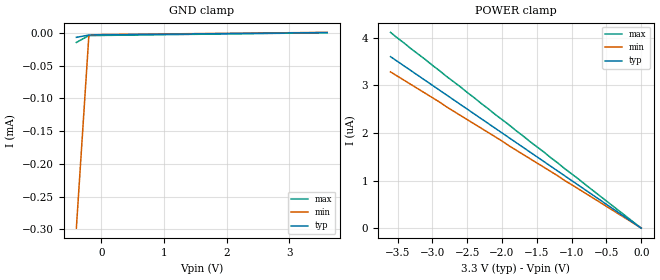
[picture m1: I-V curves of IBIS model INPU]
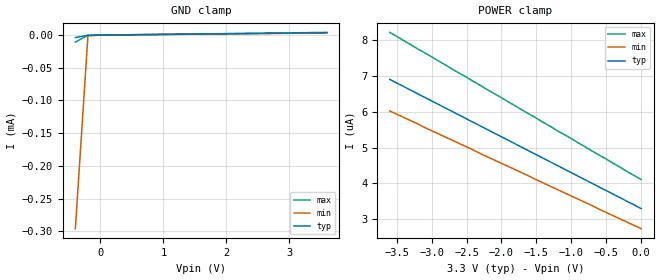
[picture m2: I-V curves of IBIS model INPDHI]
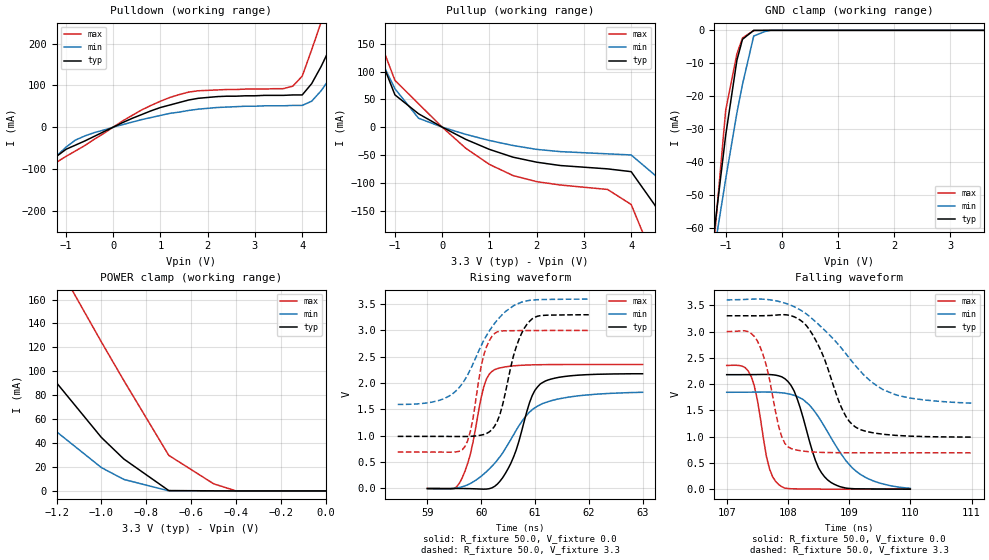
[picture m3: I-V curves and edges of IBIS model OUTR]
|   Texas Instruments Incorporated
|   Data Transmissions Products
|   IBIS Model for ISO723x4x
|   16DW SOIC Package
[IBIS Ver]   3.2
[Comment char]   |_char
[File name]   iso35.ibs
[File Rev]   1.0
[Date]   08July08
[Source]   File originated at Texas Instruments Incorporated.
   Data Transmission Products Group.
[Notes]
[Disclaimer]
(C) Copyright Texas Instruments Incorporated 2002
   All rights reserved
  Texas Instruments Incorporated hereby grants the user of this IBIS
model a non-exclusive, nontransferable license to use this IBIS model
under the following terms.  Before using this IBIS model, the user
should read this license.  If the user does not accept these terms,
the IBIS model should be returned to Texas Instruments within 30 days.
  The user is granted this license only to use the IBIS model and
is not granted rights to sell, load, rent, lease or license the IBIS
model in whole or in part, or in modified form to anyone other than
user.  User may modify the IBIS model to suit its specific applications
but rights to derivative works and such modifications shall belong to
Texas Instruments.
  This IBIS model is provided on an "AS IS" basis and Texas Instruments
makes absolutely no warranty with respect to the information contained
herein.  TEXAS INSTRUMENTS DISCLAIMS AND CUSTOMER WAIVES ALL WARRANTIES,
EXPRESS OR IMPLIED, INCLUDING WARRANTIES OF MERCHANTABILITY OR FITNESS
FOR A PARTICULAR PURPOSE. The entire risk as to quality and performance
is with the Customer. ACCORDINGLY, IN NO EVENT SHALL THE COMPANY BE LIABLE
FOR ANY DAMAGES, WHETHER IN CONTRACT OR TORT,INCLUDING ANY LOST PROFITS
OR OTHER INCIDENTAL, CONSEQUENTIAL, EXEMPLARY, OR PUNITIVE DAMAGES ARISING
OUT OF THE USE OR APPLICATION OF THE IBIS model provided in this package.
Further, Texas Instruments reserves the right to discontinue or make changes
without notice to any product herein to improve reliability, function, or
design. Texas Instruments does not convey any license under patent rights
or any other intellectual property rights, including those of third parties.
Contact Texas Instruments at ATTN:DATA TRANSMISSIONS
[Copyright]   Copyright 2002, Texas Instruments, All Rights Reserved
[Component]   ISO35DW
[Manufacturer]  Texas Instruments Incorporated
[Package]
|   typ   min   max
R_pkg   0.04817   0.03432   0.09530
L_pkg   2.4595nH   1.6904nH   4.7034nH
C_pkg   0.847pF   0.428pF   1.397pF
[Pin]   signal_name   model_name   R_pin   L_pin   C_pin
1   VCC1   POWER   0.03455  3.39778n  0.89677p
2   GND1   GND   0.03432  3.12613n  0.84706p
3   R   OUTR   0.04265  1.85523n  0.57831p
4   REB   INPU   0.03948  1.69049n  0.59300p
5   DE   INPDHI   0.03943  1.70546n  0.55709p
6   D   INPU   0.04257  1.86953n  0.56379p
7   GND1   GND   0.04783  1.99000n  0.60148p
8   GND1   GND   0.03740  4.70338n  1.39696p
9   GND2   GND   0.03763  4.61305n  1.39587p
10   GND2   GND   0.04703  2.01514n  0.58483p
11   Y   DRVR   0.07132  2.45946n  0.43321p
12   Z   DRVR   0.06147  2.13194n  0.42769p
13   B   REC   0.07288  2.39260n  0.48001p
14   A   REC   0.09530  3.03704n  0.47622p
15   GND2   GND   0.04817  4.23145n  0.93567p
16   VCC2   POWER   0.04790  4.51154n  0.99405p
[Diff_pin]   inv_pin   vdiff   tdelay_typ   tdelay_min   tdelay_max
| The 'A' pin is Diff_pin and the 'B' pin is the inv_pin
11   12   0.200   0 0 0
13   14   0.200   0 0 0
| Models and submodels in the file (5): INPU (Input), INPDHI (Input), OUTR (3-state), REC (Input), DRVR (I/O)
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|   Driver Input / Receiver Enable Model
[Model]   INPU
Model_type   Input
|Signals   REB,D
Vinh = 2.0
Vinl = 0.8
|   typ   min   max
C_comp   1.3pF   1.1pF   1.5pF
|   typ   min   max
[Temperature Range]   27   -40   85
[Voltage range]   3.3V   3.0V   3.6V
[GND_clamp]
|   Voltage   I(typ)   I(min)   I(max)
-400mV    -7.04uA    -298uA     -14.8uA
-200mV    -3.5uA     -3.91uA    -4.34uA
0V        -3.3uA     -2.74uA    -4.11uA
3.6V      300nA      549nA      14.4pA
[Power_clamp]
| Note that the[POWER_clamp]voltage table is referenced to Vcc
| and is calculated using Vtable=Vcc - Vmeasured.
|   Voltage   I(typ)   I(min)   I(max)
-3.6V     3.6uA      3.28uA     4.11uA
-2.9V     2.9uA      2.65uA     3.31uA
-2.8V     2.8uA      2.55uA     3.19uA
0V        0A         0A         0A
|   Driver Enable
[Model]   INPDHI
Model_type   Input
|Signals   DE
Vinh = 2.0
Vinl = 0.8
|   typ   min   max
C_comp   1.3pF   1.1pF   1.5pF
|   typ   min   max
[Temperature Range]   27   -40   85
[Voltage range]   3.3V   3.0V   3.6V
[GND_clamp]
|   Voltage   I(typ)   I(min)   I(max)
-400mV    -3.79uA    -296uA     -10.8uA
-200mV    -202nA     -1.2uA     -230nA
0V        0A         0A         0A
3.6V      3.6uA      3.28uA     4.11uA
[Power_clamp]
| Note that the[POWER_clamp]voltage table is referenced to Vcc
| and is calculated using Vtable=Vcc - Vmeasured.
|   Voltage   I(typ)   I(min)   I(max)
-3.6V     6.9uA      6.02uA     8.21uA
-500mV    3.8uA      3.19uA     4.68uA
-200mV    3.5uA      2.92uA     4.33uA
0V        3.3uA      2.74uA     4.11uA
[Model]   OUTR
Model_type   3-state
| Signals   R
Vmeas = 2.2V   |Reference voltage for timing measurements
Cref = 15pF   |Timing specification test load capacitance value
Vref = 0   |Timing specification test load voltage; GND
| variable   typ   min   max
C_comp   2.1pF   1.7pF   2.5pF
|   typ   min   max
[Temperature Range]   25.0   -40   85
[Voltage range]   3.3V   3.6V   3.0V
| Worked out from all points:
|   slope of the pulldown table from 0 to 0.495 V, typ, clamps not added: 19.6 ohm
|   slope of the pullup table from 0 to 0.495 V, typ, clamps not added: 22.7 ohm
|   GND clamp passes 1 mA (typ) near -0.57 V on its own axis
|   POWER clamp passes 1 mA (typ) near -0.71 V on its own axis
|   rising waveform, R_fixture 50.0, V_fixture 0.0: 20-80 % time 410ps typ, 767ps min, 290ps max; typ from 0 V to 2.18 V
|   falling waveform, R_fixture 50.0, V_fixture 0.0: 20-80 % time 345ps typ, 638ps min, 215ps max; typ from 2.18 V to 0.001 V
|   rising waveform, R_fixture 50.0, V_fixture 3.3: 20-80 % time 344ps typ, 645ps min, 237ps max; typ from 0.989 V to 3.3 V
|   falling waveform, R_fixture 50.0, V_fixture 3.3: 20-80 % time 465ps typ, 950ps min, 260ps max; typ from 3.3 V to 0.991 V
[Pulldown]
|   Voltage   I(typ)  I(min)  I(max)
-3.6V     -427mA     -334mA     -572mA
-2.8V     -304mA     -244mA     -401mA
-2.4V     -243mA     -200mA     -316mA
-2V       -182mA     -155mA     -231mA
-1.2V     -70mA      -69mA      -84mA
-400mV    -22mA      -13mA      -29mA
1.4V      59mA       36mA       78mA
3.8V      77mA       52mA       98mA
4.4V      145mA      87mA       251mA
4.8V      241mA      154mA      387mA
5.4V      390mA      263mA      593mA
7.2V      850mA      600mA      1.226A
[Pullup]
|   Voltage   I(typ)  I(min)  I(max)
| Note that the[Pullup]voltage table is referenced to Vcc
| and is calculated using Vtable=Vcc - Vmeasured.
-3.6V     689mA      544mA      913mA
-2V       288mA      247mA      363mA
-1.5V     166mA      156mA      196mA
-1V       58mA       69mA       84mA
-500mV    24mA       16mA       42mA
1.5V      -54mA      -33mA      -87mA
3.5V      -75mA      -48mA      -112mA
4V        -80mA      -50mA      -139mA
4.5V      -140mA     -86mA      -242mA
5V        -217mA     -140mA     -350mA
5.5V      -295mA     -196mA     -458mA
7.2V      -562mA     -390mA     -830mA
[GND_clamp]
|   Voltage   I(typ)   I(min)   I(max)
| Outputs in High Impedance (off)
-3.6V     -425.9mA   -334mA     -570.9mA
-1.2V     -60.51mA   -66.54mA   -62.98mA
-1.1V     -46.2mA    -55.88mA   -43.66mA
-1V       -31.9mA    -45.23mA   -24.35mA
-800mV    -9.097mA   -25.09mA   -7.168mA
-700mV    -2.72mA    -16.39mA   -2.309mA
-500mV    -16.68uA   -1.726mA   -51.55uA
-300mV    -3.339uA   -347.5uA   -10.31uA
-200mV    -4.168nA   -2.232uA   -2.942nA
3.6V      8.784nA    32.33nA    5.263uA
[POWER_clamp]
|   Voltage  I(typ)   I(min)   I(max)
| Note that the [POWER_clamp] voltage table is referenced to Vcc
| and is calculated using Vtable = Vcc - Vmeasured.
| Outputs in Tri-state.
-3.6V     688.9mA    487.5mA    1.016A
-1.9V     261.9mA    173.3mA    429.5mA
-1.8V     237.1mA    155.1mA    395.2mA
-1.5V     163.1mA    101.4mA    292.7mA
-1.2V     90.4mA     49.49mA    191mA
-1.1V     67.54mA    34.49mA    157.7mA
-1V       44.68mA    19.49mA    124.5mA
-900mV    26.67mA    9.609mA    92.23mA
-700mV    313.1uA    71.19uA    29.75mA
-500mV    62.63uA    14.3uA     5.96mA
-400mV    17.51nA    62.62nA    10.53uA
0V        50.28pA    1.949nA    141.4pA
[Ramp]
|   typ   min   max
dV/dt_r   1.88V/.33ns   1.48V/.58ns   1.81V/.23ns
dV/dt_f   1.92V/.36ns   1.67V/.60ns   2.07V/.23ns
R_load = 50
[Rising Waveform]
R_fixture = 50.0
V_fixture = 0.0
C_fixture = 0p
L_fixture = 0n
|   V(typ)   V(min)   V(max)
59ns      -7.749uV   -5.606mV   288.9uV
59.6ns    -109.3uV   19.92mV    107.1mV
59.8ns    -3.444mV   95mV       650.6mV
60.05ns   -12.83mV   275mV      1.934V
60.25ns   39.93mV    475.7mV    2.256V
60.55ns   472.4mV    926.2mV    2.323V
60.9ns    1.631V     1.452V     2.345V
61.1ns    1.985V     1.59V      2.35V
61.65ns   2.138V     1.738V     2.354V
63ns      2.178V     1.826V     2.354V
[Falling Waveform]
R_fixture = 50.0
V_fixture = 0.0
C_fixture = 0p
L_fixture = 0n
|   V(typ)   V(min)   V(max)
107ns     2.179V     1.844V     2.355V
107.4ns   2.18V      1.846V     2.146V
107.5ns   2.181V     1.847V     1.708V
107.7ns   2.181V     1.847V     384.7mV
107.9ns   2.138V     1.833V     46.95mV
108.1ns   1.873V     1.786V     6.564mV
108.4ns   547.8mV    1.458V     1.337mV
108.6ns   175.4mV    1.088V     499.6uV
109.2ns   5.764mV    269.8mV    10.24uV
110ns     850.1uV    16.75mV    -11.17uV
[Rising Waveform]
R_fixture = 50.0
V_fixture = 3.3
V_fixture_min = 3.6
V_fixture_max = 3.0
C_fixture = 0p
L_fixture = 0n
|   V(typ)   V(min)  V(max)
58.45ns   989mV      1.596V     691mV
59.3ns    989mV      1.701V     690mV
59.7ns    987mV      2.069V     798mV
59.8ns    990mV      2.26V      1.083V
60.05ns   1.025V     2.813V     2.536V
60.25ns   1.182V     3.133V     2.943V
60.4ns    1.592V     3.307V     2.992V
60.65ns   2.681V     3.494V     2.996V
60.85ns   3.115V     3.562V     2.998V
62ns      3.298V     3.596V     3V
[Falling Waveform]
R_fixture = 50.0
V_fixture = 3.3
V_fixture_min = 3.6
V_fixture_max = 3.0
C_fixture = 0p
L_fixture = 0n
|   V(typ)   V(min)  V(max)
107ns     3.3V       3.602V     3V
107.5ns   3.3V       3.618V     2.824V
107.7ns   3.303V     3.612V     2.344V
107.9ns   3.321V     3.558V     995mV
108.1ns   3.301V     3.499V     774mV
108.4ns   2.949V     3.24V      708mV
108.9ns   1.491V     2.647V     693mV
109.1ns   1.185V     2.355V     692mV
109.8ns   1.021V     1.783V     691mV
111ns     991mV      1.637V     691mV
